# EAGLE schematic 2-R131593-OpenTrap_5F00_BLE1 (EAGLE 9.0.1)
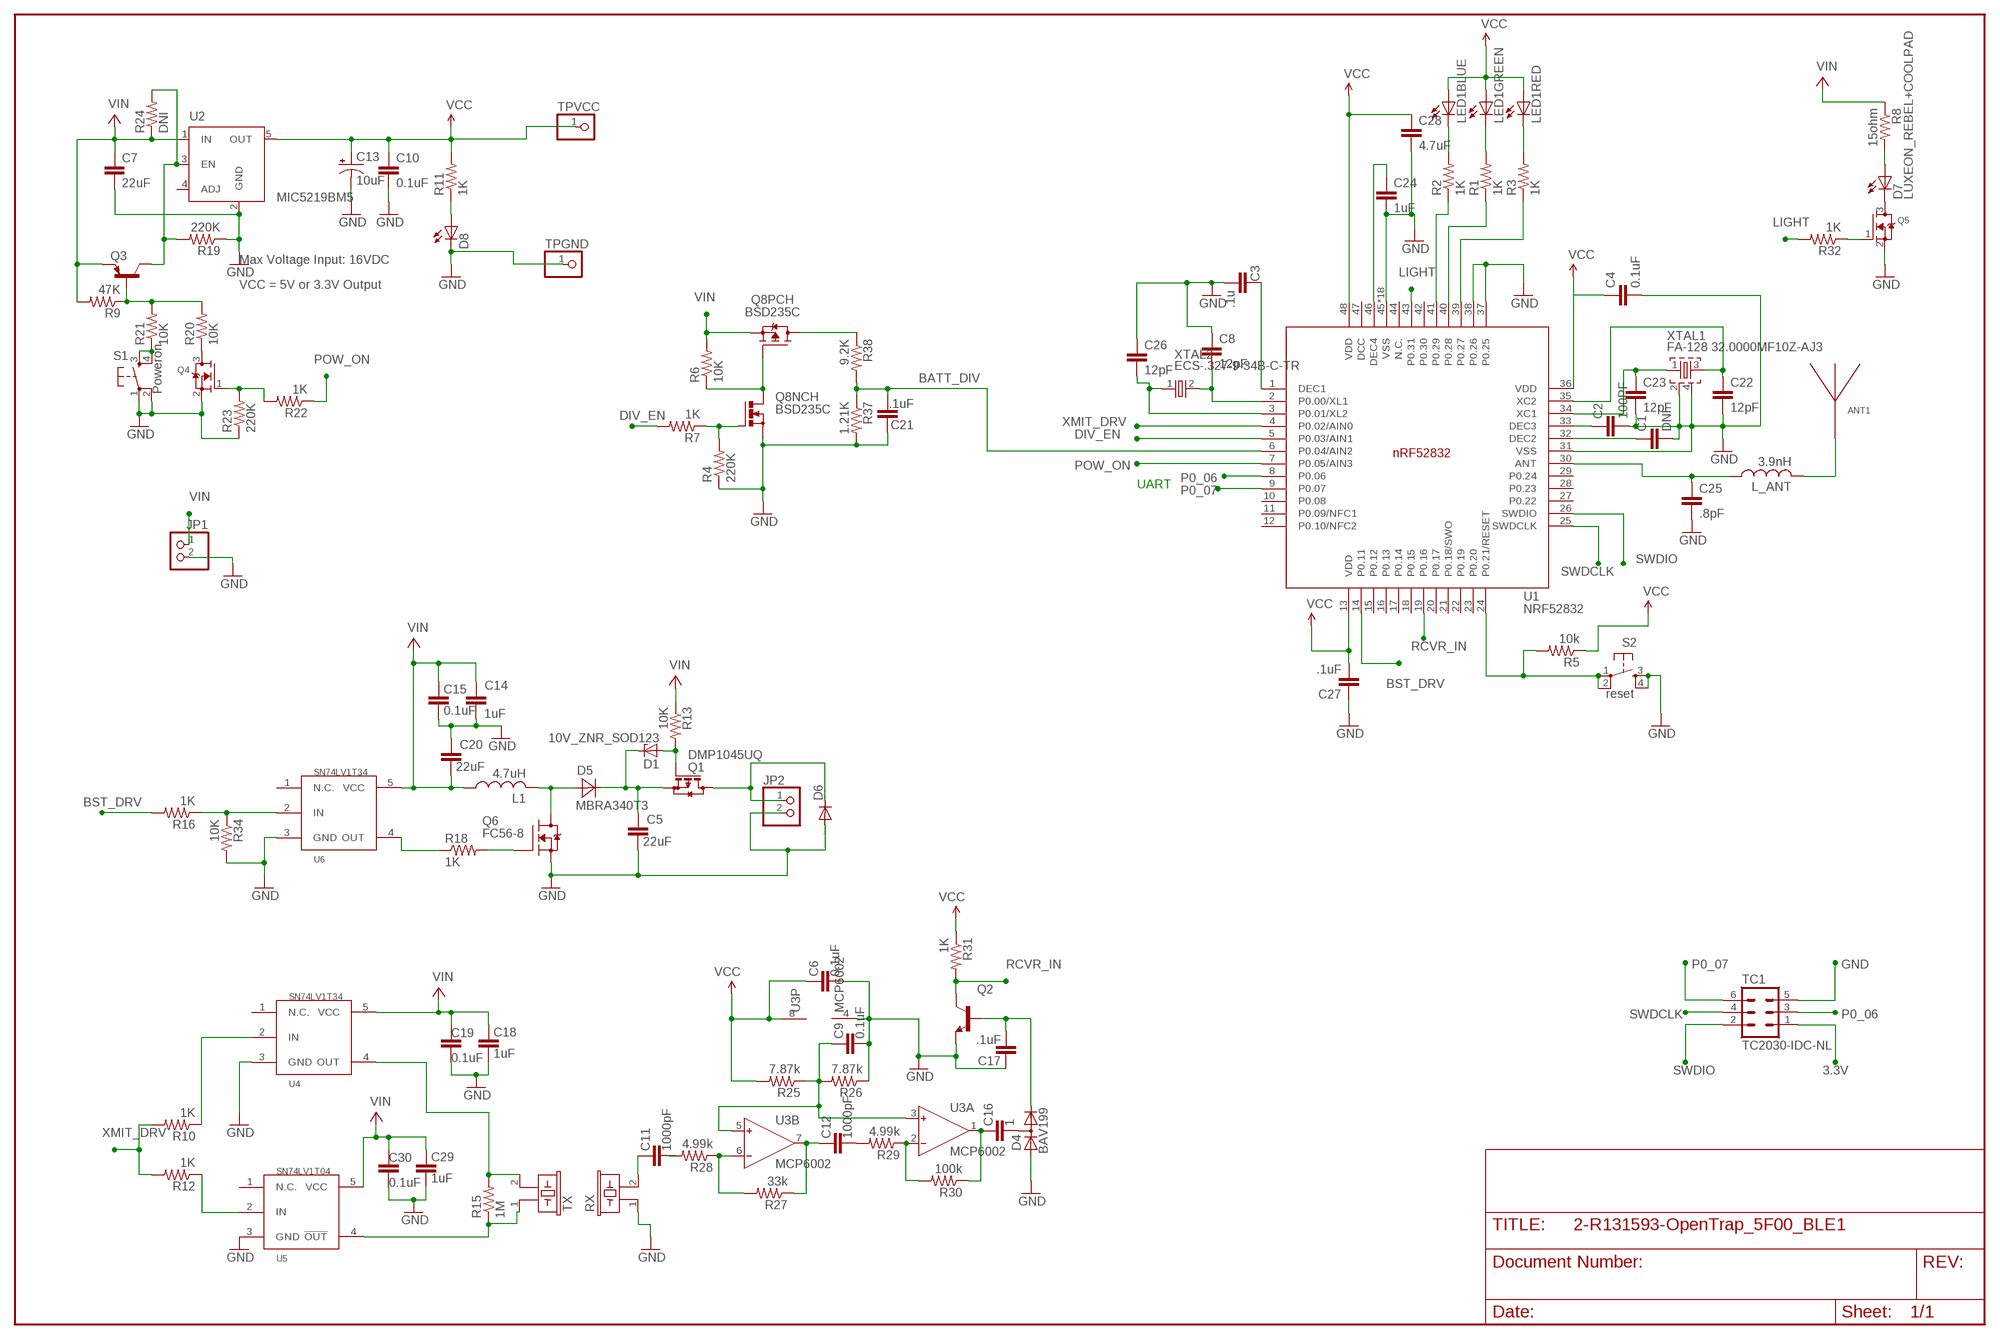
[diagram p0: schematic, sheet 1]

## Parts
ANT1  ANTENNA_QUARTER-WAVE_MONOPOLE_BEND_LEFT+1  [QWMP_BEND_LEFT_+1]
C1  DNI  C-EUC0402  [C0402]
C2  100PF  C-EUC0402  [C0402]
C3  .1u  C-EUC0402  [C0402]
C4  0.1uF  C-EUC0402  [C0402]
C5  22uF  CAP1210  [1210]
C6  0.1uF  CAP0805  [0805]
C7  22uF  C-EUC0805  [C0805]
C8  12pF  C-EUC0402  [C0402]
C9  0.1uF  CAP0805  [0805]
C10  0.1uF  CAP0805  [0805]
C11  1000pF  CAP0805  [0805]
C12  1000pF  CAP0805  [0805]
C13  10uF  CAP_POL1206  [EIA3216]
C14  1uF  CAP0805  [0805]
C15  0.1uF  CAP0805  [0805]
C16  1  CAP0805  [0805]
C17  .1uF  CAP0805  [0805]
C18  1uF  CAP0805  [0805]
C19  0.1uF  CAP0805  [0805]
C20  22uF  CAP1206  [1206]
C21  .1uF  CAP0805  [0805]
C22  12pF  C-EUC0402  [C0402]
C23  12pF  C-EUC0402  [C0402]
C24  1uF  C-EUC0603  [C0603]
C25  .8pF  C-EUC0402  [C0402]
C26  12pF  C-EUC0402  [C0402]
C27  .1uF  C-EUC0402  [C0402]
C28  4.7uF  C-EUC0603  [C0603]
C29  1uF  CAP0805  [0805]
C30  0.1uF  CAP0805  [0805]
D1  10V_ZNR_SOD123  [SOD123]
D4  BAV199  [SOT23]
D5  MBRA340T3  [SMA]
D6  DIODE-SOD123  [SOD123]
D7  LUXEON_REBEL+COOLPAD  [LUXEON_REBEL+COOLPAD]
D8  LEDCHIP-LED0805  [CHIP-LED0805]
JP1  PINHD-1X2  [1X02]
JP2  PINHD-1X2/90  [1X02/90]
L1  4.7uH  L-USV1  [ILHM2525]
L_ANT  3.9nH  INDUCTOR_0402_M  [RESC0402_M]
LED1  CLY6D-FKC  [CLY6D-FKC]
Q1  DMP1045UQ  BSS84  [SOT23]
Q2  MMBT2222ALT1-NPN-SOT23-BEC  [SOT23-BEC]
Q3  MMBT2907ALT1SMD  [SOT23-BEC]
Q4  MOSFET-NREFLOW  [SOT23]
Q5  MOSFET-NREFLOW  [SOT23]
Q6  FC56-8  [FAIRCHILD56-8]
Q8  BSD235C  [SOT363]
R1  1K  RESISTOR0402-RES  [0402-RES]
R2  1K  RESISTOR0402-RES  [0402-RES]
R3  1K  RESISTOR0402-RES  [0402-RES]
R4  220K  RESISTOR0805-RES  [0805]
R5  10k  RESISTOR0805-RES  [0805]
R6  10K  RESISTOR0805-RES  [0805]
R7  1K  RESISTOR0805-RES  [0805]
R8  15ohm  R-US_R1210  [R1210]
R9  47K  RESISTOR0805-RES  [0805]
R10  1K  RESISTOR0805-RES  [0805]
R11  1K  RESISTOR0805-RES  [0805]
R12  1K  RESISTOR0805-RES  [0805]
R13  10K  RESISTOR0805-RES  [0805]
R15  1M  RESISTOR0805-RES  [0805]
R16  1K  RESISTOR0805-RES  [0805]
R18  1K  RESISTOR0805-RES  [0805]
R19  220K  RESISTOR0805-RES  [0805]
R20  10K  RESISTOR0805-RES  [0805]
R21  10K  RESISTOR0805-RES  [0805]
R22  1K  RESISTOR0805-RES  [0805]
R23  220K  RESISTOR0805-RES  [0805]
R24  DNI  RESISTOR0805-RES  [0805]
R25  7.87k  RESISTOR0805-RES  [0805]
R26  7.87k  RESISTOR0805-RES  [0805]
R27  33k  RESISTOR0805-RES  [0805]
R28  4.99k  RESISTOR0805-RES  [0805]
R29  4.99k  RESISTOR0805-RES  [0805]
R30  100k  RESISTOR0805-RES  [0805]
R31  1K  RESISTOR0805-RES  [0805]
R32  1K  RESISTOR0805-RES  [0805]
R34  10K  RESISTOR0805-RES  [0805]
R37  1.21K  RESISTOR0805-RES  [0805]
R38  9.2K  RESISTOR0805-RES  [0805]
RX  EFBAA40D101  [EFBAA40D101]
S1  Poweron  TAC_SWITCHSMD  [TACTILE_SWITCH_SMD]
S2  reset  TAC_SWITCHSMD  [TACTILE_SWITCH_SMD]
TC1  TC2030-IDC-NL  [TC2030-IDC-NL]
TPGND  PINHD-1X1  [1X01]
TPVCC  PINHD-1X1  [1X01]
TX  EFBAA40D101  [EFBAA40D101]
U1  NRF52832  [QFN40P600X600X90-48_N]
U2  MIC5219BM5  [SOT23-5]
U3  MCP6002  AD8656RM  [MSOP08]
U4  SN74LV1T34  [SOT23-DBV]
U5  SN74LV1T04  [SOT23-DBV]
U6  SN74LV1T34  [SOT23-DBV]
XTAL1  FA-128 32.0000MF10Z-AJ3  XTAL_32MHZ  [BT-XTAL_2016_N]
XTAL2  ECS-.327-9-34B-C-TR  XTAL_32KHZ  [XTAL_3215_N]

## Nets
3.3V [vcc]: C4.1 C6.2 C10.1 C13.A(+) C27.2 C28.1 LED1.P$4(RED:A) LED1.P$5(GREEN:A) LED1.P$6(BLUE:A) R5.1 R11.2 R25.2 R31.1 TC1.1 TPVCC.1 U1.13(VDD) U1.36(VDD) U1.48(VDD) U2.5(OUT) U3.8(P:V+) ; supply symbol labelled VCC
BATT_DIV [GPIO]: C21.1 R37.1 R38.2 U1.6(P0.04/AIN2)
BST_DRV: R16.2 U1.14(P0.11)
DIV_EN [GPIO]: R7.2 U1.5(P0.03/AIN1)
EN_PLDN [GPIO]: Q3.B R9.1 R20.2 R21.2
GND [vcc]: C1.2 C2.2 C3.2 C4.2 C5.1 C6.1 C7.2 C8.1 C9.1 C10.2 C13.C(-) C14.1 C15.1 C17.2 C18.1 C19.1 C20.2 C21.2 C22.2 C23.2 C24.2 C25.2 C26.1 C27.1 C28.2 C29.1 C30.1 D4.1(A) D6.A D8.C JP1.2 JP2.2 Q2.E Q4.2(S) Q5.2(S) Q6.1(S) Q6.2(S) Q6.3(S) Q8.P$1(NCH:S) R4.1 R19.1 R23.1 R26.1 R34.2 R37.2 RX.1 S1.1 S1.2 S2.3 S2.4 TC1.5 TPGND.1 U1.31(VSS) U1.37(P0.25) U1.38(P0.26) U1.45(VSS) U1.PAD(VSS) U1.PAD@VIA01(VSS) U1.PAD@VIA02(VSS) U1.PAD@VIA03(VSS) U1.PAD@VIA04(VSS) U1.PAD@VIA05(VSS) U1.PAD@VIA06(VSS) U1.PAD@VIA07(VSS) U1.PAD@VIA08(VSS) U1.PAD@VIA09(VSS) U1.PAD@VIA10(VSS) U1.PAD@VIA11(VSS) U1.PAD@VIA12(VSS) U1.PAD@VIA13(VSS) U1.PAD@VIA14(VSS) U1.PAD@VIA15(VSS) U1.PAD@VIA16(VSS) U2.2(GND) U3.4(P:V-) U4.3(GND) U5.3(GND) U6.3(GND) XTAL1.2 XTAL1.4
LDO_EN [GPIO]: Q3.C R19.2 R24.2 U2.3(EN)
LIGHT: R32.2 U1.43(P0.31)
N$1 [GPIO]: C22.1 U1.35(XC2) XTAL1.3
N$2 [GPIO]: C23.1 U1.34(XC1) XTAL1.1
N$3 [GPIO]: R18.1 U6.4(OUT)
N$4 [GPIO]: C1.1 U1.32(DEC2)
N$5 [GPIO]: C2.1 U1.33(DEC3)
N$6 [GPIO]: R16.1 R34.1 U6.2(IN)
N$7 [GPIO]: C8.2 U1.2(P0.00/XL1) XTAL2.2
N$8: Q6.4(G) R18.2
N$9 [GPIO]: C3.1 U1.1(DEC1)
N$10 [GPIO]: C26.2 U1.3(P0.01/XL2) XTAL2.1
N$11 [GPIO]: Q8.P$5(PCH:G) Q8.P$6(NCH:D) R6.1
N$12 [GPIO]: R15.1 TX.1 U5.4(!OUT)
N$13 [GPIO]: R5.2 S2.1 S2.2 U1.24(P0.21/RESET)
N$14 [GPIO]: R15.2 TX.2 U4.4(OUT)
N$15: R3.1 U1.39(P0.27)
N$16: C11.2 RX.2
N$17 [GPIO]: C9.2 R25.1 R26.2 U3.3(A:IN+) U3.5(B:IN+)
N$18: C11.1 R28.2
N$19 [GPIO]: R12.1 U5.2(IN)
N$20: D7.C D7.C@1(C) Q5.3(D)
N$21: C12.1 R29.2
N$22: Q5.1(G) R32.1
N$23: R1.1 U1.40(P0.28)
N$24 [boost]: D7.A D7.A@1(A) R8.2
N$25: R2.1 U1.41(P0.29)
N$26: LED1.P$3(RED:C) R3.2
N$27: R21.1 S1.3 S1.4
N$28 [GPIO]: R27.2 R28.1 U3.6(B:IN-)
N$29: Q4.3(D) R20.1
N$30: LED1.P$2(GREEN:C) R1.2
N$31 [GPIO]: C12.2 R27.1 U3.7(B:OUT)
N$32 [GPIO]: Q4.1(G) R22.2 R23.2
N$33 [GPIO]: C16.2 R30.1 U3.1(A:OUT)
N$34 [GPIO]: R29.1 R30.2 U3.2(A:IN-)
N$35 [GPIO]: D6.C JP2.1 Q1.3(D)
N$36: C16.1 D4.3(AC)
N$37: LED1.P$1(BLUE:C) R2.2
N$38: D8.A R11.1
N$39 [GPIO]: R10.1 U4.2(IN)
N$41 [GPIO]: C17.1 D4.2(C) Q2.B
N$42 [GPIO]: C5.2 D1.C D5.C Q1.2(S)
N$43: C24.1 U1.46(DEC4)
N$44 [boost]: D5.A L1.2 Q6.5-8(D)
N$45 [GPIO]: D1.A Q1.1(G) R13.2
N$49 [vcc]: C25.1 L_ANT.1 U1.30(ANT)
N$50 [vcc]: ANT1.P$1 L_ANT.2
N$51: Q8.P$2(NCH:G) R4.2 R7.1
N$53: Q8.P$3(PCH:D) R38.1
P0_06 [GPIO]: TC1.3 U1.8(P0.06)
P0_07 [GPIO]: TC1.6 U1.9(P0.07)
POW_ON [GPIO]: R22.1 U1.7(P0.05/AIN3)
RCVR_IN: Q2.C R31.2 U1.19(P0.16)
SWDCLK [GPIO]: TC1.4 U1.25(SWDCLK)
SWDIO [GPIO]: TC1.2 U1.26(SWDIO)
VIN [boost]: C7.1 C14.2 C15.2 C18.2 C19.2 C20.1 C29.2 C30.2 JP1.1 L1.1 Q3.E Q8.P$4(PCH:S) R6.2 R8.1 R9.2 R13.1 R24.1 U2.1(IN) U4.5(VCC) U5.5(VCC) U6.5(VCC)
XMIT_DRV [GPIO]: R10.2 R12.2 U1.4(P0.02/AIN0)
Unconnected: U1.10(P0.08) U1.11(P0.09/NFC1) U1.12(P0.10/NFC2) U1.15(P0.12) U1.16(P0.13) U1.17(P0.14) U1.18(P0.15) U1.20(P0.17) U1.21(P0.18/SWO) U1.22(P0.19) U1.23(P0.20) U1.27(P0.22) U1.28(P0.23) U1.29(P0.24) U1.42(P0.30) U1.44(N.C.) U1.47(DCC) U2.4(ADJ) U4.1(N.C.) U5.1(N.C.) U6.1(N.C.)

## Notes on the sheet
- Max Voltage Input: 16VDC
- VCC = 5V or 3.3V Output
- UART

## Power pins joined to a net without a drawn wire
TH: D7.TH D7.TH@1(TH) D7.TH@2(TH) D7.TH@3(TH) D7.TH@4(TH) D7.TH@5(TH) D7.TH@6(TH) D7.TH@7(TH) D7.TH@8(TH) D7.TH@9(TH) D7.TH@10(TH) D7.TH@11(TH) D7.TH@12(TH) D7.TH@13(TH) D7.TH@14(TH) D7.TH@15(TH) D7.TH@16(TH) D7.TH@17(TH) D7.TH@18(TH) D7.TH@19(TH) D7.TH@20(TH) D7.TH@21(TH) D7.TH@22(TH) D7.TH@23(TH) D7.TH@24(TH) D7.TH@25(TH) D7.TH@26(TH) D7.TH@27(TH) D7.TH@28(TH) D7.TH@29(TH) D7.TH@30(TH) D7.TH@31(TH) D7.TH@32(TH) D7.TH@33(TH) D7.TH@34(TH) D7.TH@35(TH)

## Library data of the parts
ANT1 = Nordic_misc:ANTENNA_QUARTER-WAVE_MONOPOLE_BEND_LEFT
C1 C4 C24 C27 C28 = rcl:C-EU: CAPACITOR, European symbol; SPICEPREFIX: C
C2 C8 C23 C25 C26 = rcl:C-EU: CAPACITOR, European symbol; DIEL: C0G; SPICEPREFIX: C
C3 = rcl:C-EU: CAPACITOR, European symbol; DIEL: x7r; SPICEPREFIX: C
C5 C6 C9-C12 C14-C21 C29 C30 = SparkFun:CAP: Capacitor
C7 = rcl:C-EU: CAPACITOR, European symbol
C13 = SparkFun:CAP_POL: Capacitor Polarized
C22 = rcl:C-EU: CAPACITOR, European symbol; DIEL: c0g; SPICEPREFIX: C
D1 = Roger_lib:10V_ZNR_SOD123
D4 = diode:BAV199: DIODE low-leakage double diode
D5 = diode:MBRA340T3: Surface Mount Schottky Power Rectifier
D6 = diode:DIODE-: DIODE
D7 = led-lumiled:LUXEON_REBEL+COOLPAD: LUXEON REBEL LED with cooling pads Display Layer Refence in Board for more information Stop and Cream Mask defined by Luxeon Rebel Footprint _customer.dxf; OC_FARNELL: unknown; OC_NEWARK: unknown
D8 = led:LED: LED
JP1 JP2 = pinhead:PINHD-1X2: PIN HEADER
L1 = Rogerlib:L-US: INDUCTOR, American symbol
L_ANT = Nordic_nRF:INDUCTOR: Generic chip inductor
LED1 = Roger_lib:CLY6D-FKC
Q1 = transistor-small-signal:BSS84: P-CHANNEL MOS FET
Q2 = transistor-neu-to92:*-NPN-: NPN Transistror
Q3 = transistor-pnp:MMBT2907*: PNP Transistror
Q4 Q5 = adafruit:MOSFET-N: N-Channel Mosfet 2N7002E - 60V 260mA SOT23 [Digikey: 2N7002ET1GOSTR-ND] - REEL BSH103 - 30V 850mA SOT23 [Digikey: 568-5013-1-ND]
Q6 = testlibFC56-8:FC56-8
Q8 = Roger_lib:BSD235C: Dual N-P Channel
R1-R7 R9-R13 R15 R16 R18-R32 R34 R37 R38 = SparkFun:RESISTOR: Resistor
R8 = rcl:R-US_: RESISTOR, American symbol
RX TX = buzzer:EFB?: Piezoelectric Acoustic Transducer; OC_FARNELL: unknown; OC_NEWARK: unknown
S1 S2 = SparkFun:TAC_SWITCH: Momentary Switch Button commonly used for reset or general input. Spark Fun Electronics SKU : COM-00097
TC1 = TagConnect:TC2030-IDC: Tag-Connect In Circuit Programming & Debug Cable 6 Pin http://www.tag-connect.com
TPGND TPVCC = pinhead:PINHD-1X1: PIN HEADER
U1 = Nordic_nRF:NRF52832: nRF52832 Features Single chip, highly flexible, 2.4 GHz multi-protocol SoC 32-bit ARM Cortex-M4F Processor 1.7v to 3.6v operation 512kB flash + 64kB RAM Supports concurrent Bluetooth Smart/ANT protocol operation On-chip NFC tag for Out-of-Band (OOB) pairing Up to +4dBm output power -96dBm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
U2 = v-reg-micrel:MIC5219BM5: VOLTAGE REGULATOR; MF: ALTERA CORPORATION; MPN: MIC5219BM5 TR; OC_FARNELL: 1100656; OC_NEWARK: 09J8939
U3 = analog-devices:AD8656: Low Noise, Precision CMOS Amplifier Source: http://www.analog.com/static/imported-files/data_sheets/AD8655_8656.pdf; MPN: AD8656ARMZ; OC_FARNELL: 1117887; OC_NEWARK: 34P3252
U4 U6 = Roger_lib:SN74LV1T34
U5 = Roger_lib:SN74LV1T04
XTAL1 = Nordic_nRF:XTAL_32MHZ
XTAL2 = Nordic_nRF:XTAL_32KHZ

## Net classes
1 vcc: width 0.254 mm
2 GPIO: width 0.152 mm
3 boost: width 0.381 mm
